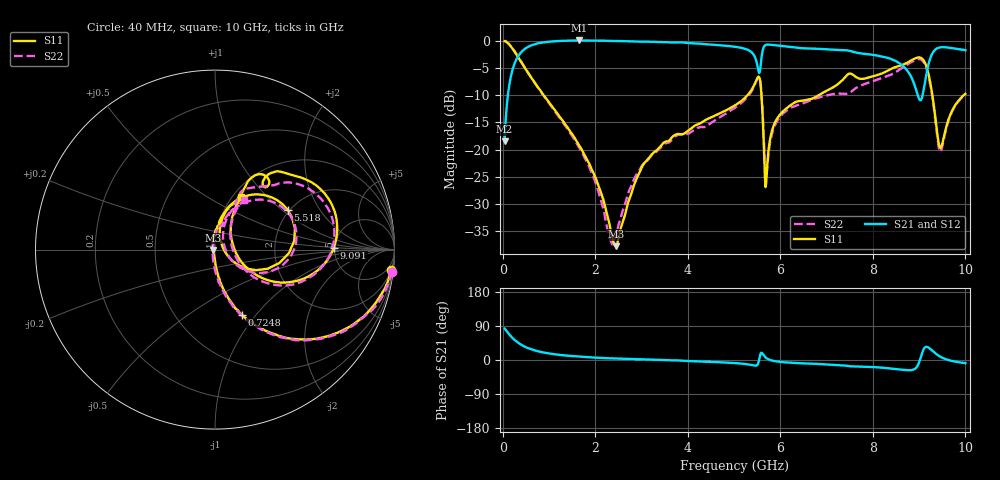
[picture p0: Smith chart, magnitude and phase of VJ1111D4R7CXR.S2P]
! VJ1111D4R7CXR
! DATE 03/04/2022  14:17
! CAPACITORS MOUNTED IN SERIES ON 25 MIL THICK MICROSTRIP SUBSTRATE
# GHz  S  MA  R  50.00
!  FREQ  S11M  S11A  S21M  S21A  S12M  S12A  S22M  S22A
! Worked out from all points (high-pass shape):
!   801 points, 40 MHz to 10 GHz, reference 50 ohm
!   highest |S21| = 0.01 dB at 1.646 GHz (marker M1); lowest = -18.5 dB at 40 MHz (marker M2)
!   |S21| within 3 dB of the highest: 325.3 MHz to 5.448 GHz (5.123 GHz wide, 177 % of centre); 5.596 GHz to 8.229 GHz (2.633 GHz wide, 38.1 % of centre)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
!   lowest |S11| = -37.7 dB at 2.443 GHz (marker M3), VSWR 1.03, Z = 48.7 - j0.155 ohm
!   |S11| at or under -10 dB: 880.8 MHz to 5.295 GHz (4.414 GHz wide, 143 % of centre); 5.592 GHz to 6.838 GHz (1.246 GHz wide, 20 % of centre); 9.285 GHz to 9.967 GHz (681.6 MHz wide, 7.08 % of centre)
!   |S22| runs from -37.4 to 0.0 dB; largest |S21 - S12| = 0.0085
!   S11 on the Smith chart (normalised r, x): 40 MHz: 2, -17; 724.8 MHz: 0.99, -0.85; 5.518 GHz: 1.95, +1.10; 9.091 GHz: 4.93, +0.18; 10 GHz: 1.09, +0.71
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0.04  0.9865 -6.7  0.119 82.9  0.1192 82.9  0.9958 -7.1
0.25165  0.7959 -37.2  0.6092 53.4  0.6097 53.3  0.8008 -37.2
0.72475  0.3914 -67.8  0.9325 24.3  0.9363 24.2  0.3893 -68.4
1.64605  0.1102 -85.7  1.001 8.9  1.005 8.8  0.1053 -91.1
1.7083  0.09941 -86.4  1.001 8.4  1.006 8.3  0.0946 -92.4
2.3308  0.01843 -118.3  0.9914 4.4  0.9964 4.2  0.01457 -165.3
2.44285  0.01299 -173.0  0.9893 4.0  0.9932 3.8  0.0166 136.8
2.86615  0.05096 106.0  0.978 2.1  0.9826 2.0  0.05653 97.8
3.36415  0.1017 89.3  0.9662 0.2  0.9705 0.1  0.09933 85.9
5.02  0.2541 71.5  0.8759 -8.1  0.8799 -8.3  0.2421 65.8
5.518  0.462 28.6  0.5509 -9.9  0.5537 -10.0  0.4607 24.4
5.60515  0.256 -26.7  0.7574 18.1  0.7609 17.9  0.2717 -29.0
5.65495  0.07862 -26.0  0.8887 10.0  0.8927 9.8  0.09705 -30.1
5.70475  0.05945 58.5  0.9156 4.5  0.9197 4.3  0.05983 35.9
5.9413  0.1954 76.0  0.8986 -4.2  0.902 -4.3  0.1856 69.1
6.6883  0.293 65.2  0.8418 -9.7  0.8457 -9.9  0.2862 66.3
8.34415  0.5343 53.4  0.688 -21.8  0.6919 -21.9  0.4777 48.5
8.84215  0.6616 33.7  0.4505 -26.5  0.4532 -26.7  0.6387 29.7
9.09115  0.6629 0.9  0.3409 26.9  0.343 26.7  0.6397 -2.9
9.24055  0.4116 -26.5  0.687 29.4  0.6897 29.1  0.393 -30.2
9.4522  0.1041 11.1  0.8646 9.0  0.8687 8.9  0.09545 10.1
10  0.3243 63.9  0.8148 -8.2  0.8188 -8.4  0.3197 59.8
